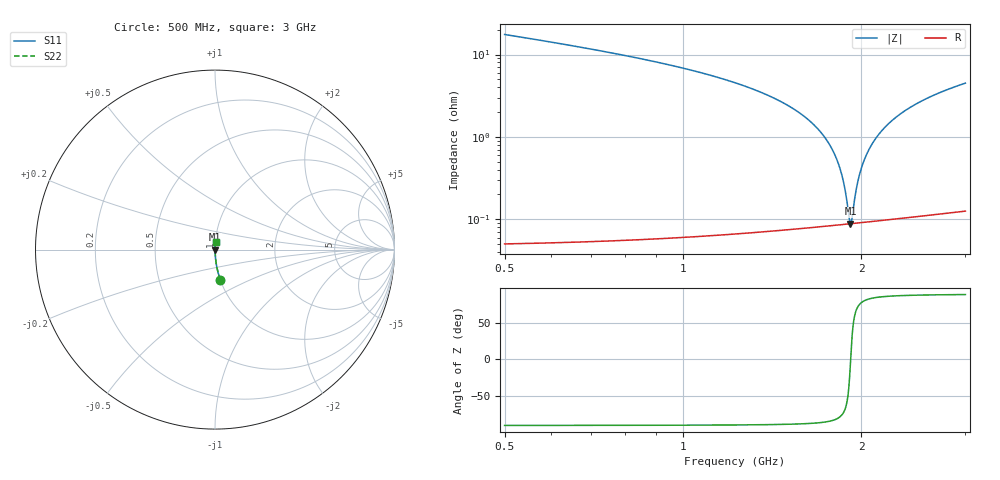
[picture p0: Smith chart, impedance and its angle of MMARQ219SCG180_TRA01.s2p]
! MMARQ219SCG180_TRA01  S-PARAMETER MODEL  ( General Type )
! Model Generated by TAIYO YUDEN Corporation (http://www.ty-top.com)
! Version 1.0
! TAIYO YUDEN Control No. 150609
! Copyright(c) 2015 TAIYO YUDEN CO.,LTD. All Rights Reserved.
! Product Description (link to TY-COMPAS)
! https://ds.yuden.co.jp/TYCOMPAS/or/detail?pn=MMARQ219SCG180JTRA01&u=M
! Products Name : Multilayer Ceramic Capacitors
! Characteristics :
!  Capacitance : 18 pF , Rated Voltage : 250V , TCC : CG / C0G
!  Case Size : 2.0 x 1.25 / 0.079 x 0.049 [mm/inch] , Thickness : 0.85 / 0.033 [mm/inch]
!  (Conditions: Temperature = 25 degC , DC Bias Current/Voltage = 0A / 0V)
! External Node Assignments :
!  1  o---| |---o  2
! GND o---------o GND
! Frequency Range : 500MHz  -  3GHz  [ 401 STEP ]
# MHz S RI R 50
! Freq[MHz].  S11 Real  S11 Imag  S21 Real  S21 Imag  S12 Real  S12 Imag  S22 Real  S22 Imag
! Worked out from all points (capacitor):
!   401 points, 500 MHz to 3 GHz, reference 50 ohm
!   read as one part in series: C = 16.9 pF near 512.5 MHz
!   lowest |Z| = 88.4 mohm at 1.919 GHz (marker M1)
!   series resonance near 1.92 GHz, so ESL is about 410 pH
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500  0.0302 -0.1697  0.9698 0.1697  0.9698 0.1697  0.0302 -0.1697
918.75  0.00674 -0.0782  0.9933 0.0782  0.9933 0.0782  0.00674 -0.0782
1337.5  0.00199 -0.036  0.998 0.036  0.998 0.036  0.00199 -0.036
1587.5  0.00112 -0.0187  0.9989 0.0187  0.9989 0.0187  0.00112 -0.0187
1675  0.000978 -0.0134  0.999 0.0134  0.999 0.0134  0.000978 -0.0134
1750  0.000906 -0.00905  0.9991 0.00905  0.9991 0.00905  0.000906 -0.00905
1800  0.00088 -0.0063  0.9991 0.0063  0.9991 0.0063  0.00088 -0.0063
1843.75  0.000871 -0.00395  0.9991 0.00395  0.9991 0.00395  0.000871 -0.00395
1868.75  0.000871 -0.00264  0.9991 0.00264  0.9991 0.00264  0.000871 -0.00264
1881.25  0.000872 -0.00199  0.9991 0.00199  0.9991 0.00199  0.000872 -0.00199
1906.25  0.000877 -0.000706  0.9991 0.000706  0.9991 0.000706  0.000877 -0.000706
1918.75  0.00088 -6.91e-05  0.9991 6.91e-05  0.9991 6.91e-05  0.00088 -6.91e-05
1931.25  0.000885 0.000563  0.9991 -0.000563  0.9991 -0.000563  0.000885 0.000563
1956.25  0.000896 0.00182  0.9991 -0.00182  0.9991 -0.00182  0.000896 0.00182
1975  0.000907 0.00275  0.9991 -0.00275  0.9991 -0.00275  0.000907 0.00275
2012.5  0.000933 0.00458  0.9991 -0.00458  0.9991 -0.00458  0.000933 0.00458
2043.75  0.00096 0.00608  0.999 -0.00608  0.999 -0.00608  0.00096 0.00608
2081.25  0.000997 0.00785  0.999 -0.00785  0.999 -0.00785  0.000997 0.00785
2168.75  0.00111 0.0119  0.9989 -0.0119  0.9989 -0.0119  0.00111 0.0119
2343.75  0.00141 0.0195  0.9986 -0.0195  0.9986 -0.0195  0.00141 0.0195
2587.5  0.00198 0.0294  0.998 -0.0294  0.998 -0.0294  0.00198 0.0294
3000  0.00326 0.0447  0.9967 -0.0447  0.9967 -0.0447  0.00326 0.0447
